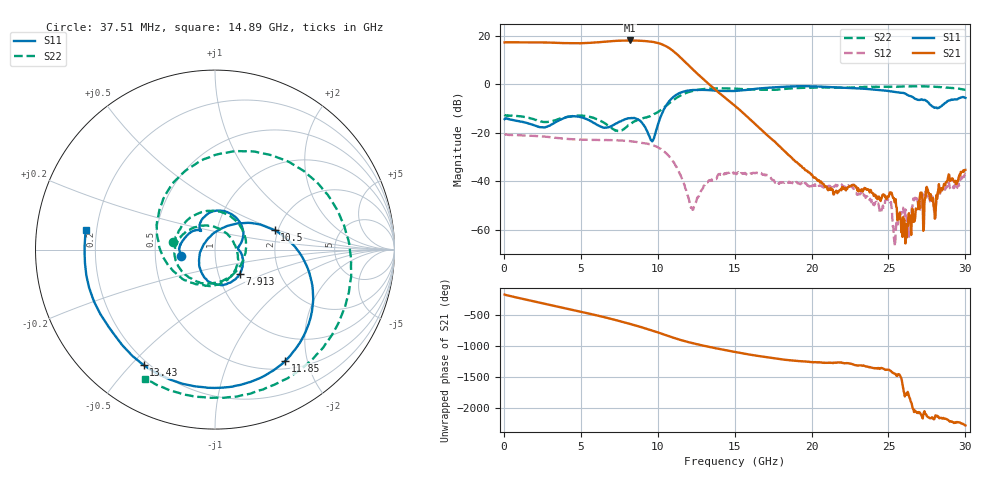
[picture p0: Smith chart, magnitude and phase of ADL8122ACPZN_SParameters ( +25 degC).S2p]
! "Analog Devices, Inc."
! Device:	ADL8122ACPZN
! Description:	"10 kHz to 10 GHz, Wideband, Low Noise Amplifier"
! Conditions:	Vdd = 5.0 V
!		IDQ = 95 mA
!		Pin = -25 dBm
!		Operating Temperature = +25 C (at package bottom)
! Product validation unit SN1 soldered down to Evaluation Board as shown on ADL8122-EVALZ User Guide. Board loss de-embedded from S21 magnitude.  All other RF measurements reference to RF coaxial connector.
! Frequency (GHz)	S11_Mag (dB)	S11_Phase (deg)	S21_Mag (dB)	S21_Phase (deg)	S12_Mag (dB)	S12_Phase (deg)	S22_Mag (dB)	S22_Phase (deg)
#  GHZ  S  DB  R 50
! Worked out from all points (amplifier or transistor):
!   800 points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, 37.51 MHz to 30 GHz, reference 50 ohm
!   highest |S21| = 18.1 dB at 8.175 GHz (marker M1)
!   |S21| within 3 dB of that: start of sweep to 10.7 GHz
!   unconditionally stable (mu >= 1): start of sweep to end of sweep
!   at 5.025 GHz: K = 1.18, MAG = 17.3 dB, |S12| = -22.8 dB
!   at 15.04 GHz: K = 14.28, MAG = -0.8 dB, |S12| = -36.5 dB
!   at 30 GHz: K = 612.24, MAG = -29.9 dB, |S12| = -37.2 dB
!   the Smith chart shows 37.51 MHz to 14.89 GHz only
!   S11 on the Smith chart (normalised r, x): 37.51 MHz: 0.68, -0.05; 7.913 GHz: 1.27, -0.35; 10.5 GHz: 1.92, +0.47; 11.85 GHz: 0.61, -1.64; 13.43 GHz: 0.18, -0.54; 14.89 GHz: 0.16, +0.07
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0.03750899  -14.34 -168.6  17.26 -178.3  -20.86 1.6  -12.48 169.8
0.9000087  -15.11 154.1  17.30 129.9  -20.95 -43.7  -13.08 114.7
1.575009  -16.10 137.8  17.28 92.5  -21.13 -76.2  -13.76 67.2
3.037508  -16.72 126.0  17.18 11.3  -21.77 -148.0  -15.27 -59.8
3.900008  -13.91 102.3  16.98 -35.2  -22.34 169.8  -13.73 -123.5
5.062508  -13.65 50.2  16.95 -97.3  -22.76 112.9  -12.90 -173.7
5.775007  -15.65 21.4  17.16 -136.8  -22.88 76.5  -13.80 160.5
6.600007  -17.87 3.3  17.58 174.9  -22.95 32.3  -16.17 121.2
7.200007  -16.39 -10.3  17.88 137.7  -23.03 -1.3  -18.92 68.6
7.912507  -14.29 -43.8  18.06 90.8  -23.27 -42.1  -17.80 -11.5
8.175007  -13.98 -58.8  18.07 73.1  -23.39 -57.8  -16.44 -34.7
9.150006  -17.44 -128.5  17.84 3.8  -24.28 -117.0  -13.73 -99.6
10.05001  -15.68 56.8  16.94 -67.5  -26.09 -179.7  -11.19 -161.6
10.50001  -9.13 17.9  15.80 -105.6  -28.21 145.5  -9.04 157.0
11.06251  -4.94 -18.2  13.42 -152.7  -32.41 101.3  -6.25 103.2
11.85001  -2.70 -57.8  8.79 150.0  -43.77 35.7  -3.54 38.9
13.425  -2.43 -121.8  -0.47 60.2  -39.77 168.8  -1.72 -53.5
14.8875  -2.77 171.5  -8.19 -10.1  -36.27 100.7  -1.75 -118.4
15.0375  -2.71 164.5  -8.98 -16.9  -36.46 96.0  -1.80 -124.8
20.025  -0.81 16.0  -37.22 -178.8  -42.03 -56.0  -1.41 49.4
25.0125  -2.75 -118.3  -46.31 60.8  -47.22 111.0  -1.02 -102.7
30  -5.60 -104.3  -35.24 -111.6  -37.16 -115.2  -2.26 -160.6
